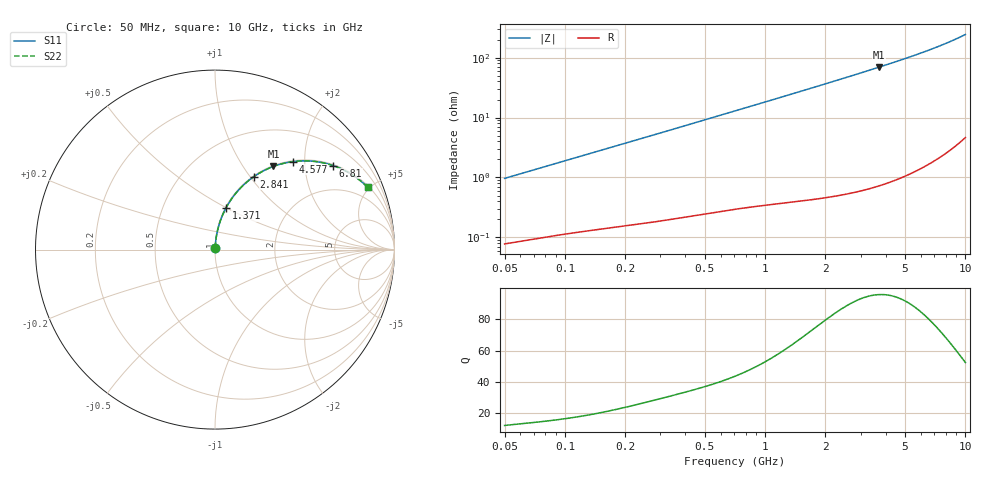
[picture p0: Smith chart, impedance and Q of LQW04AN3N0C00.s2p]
!Murata Part Number: LQW04AN3N0C00
!These Parameters are Measured in Series Mode Connection
!  o--[Z]--o
!Port1  Port2
!  o-------o
!Freq. Start=50[MHz] Stop=10[GHz], 401[Steps]
# Hz S RI R 50
!Freq.(Hz)	S 11(Real)	S 11(Imag)	S 21(Real)	S 21(Imag)	S 12(Real)	S 12(Imag)	S 22(Real)	S 22(Imag)
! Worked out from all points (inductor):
!   401 points, 50 MHz to 10 GHz, reference 50 ohm
!   read as one part in series: L = 3.04 nH near 51.34 MHz
!   highest Q = 95.6 at 3.703 GHz (marker M1), where L = 2.97 nH
!   S11 on the Smith chart (normalised r, x): 50 MHz: 1.00, +0.02; 1.371 GHz: 1.01, +0.50; 2.841 GHz: 1.01, +1.05; 4.577 GHz: 1.02, +1.74; 6.81 GHz: 1.04, +2.79; 10 GHz: 1.09, +4.86
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5e7  0.000871 0.00961  0.9991 -0.00961  0.9991 -0.00961  0.000871 0.00961
5.134228e7  0.000887 0.00986  0.9991 -0.00986  0.9991 -0.00986  0.000887 0.00986
1.214486e8  0.00176 0.0227  0.9982 -0.0227  0.9982 -0.0227  0.00176 0.0227
1.956524e8  0.00284 0.0361  0.9972 -0.0361  0.9972 -0.0361  0.00284 0.0361
2.949953e8  0.00479 0.054  0.9952 -0.054  0.9952 -0.054  0.00479 0.054
4.689809e8  0.00964 0.0848  0.9904 -0.0848  0.9904 -0.0848  0.00964 0.0848
7.071068e8  0.0191 0.126  0.9809 -0.126  0.9809 -0.126  0.0191 0.126
9.978194e8  0.0349 0.1744  0.9651 -0.1744  0.9651 -0.1744  0.0349 0.1744
1.371241e9  0.0617 0.2329  0.9383 -0.2329  0.9383 -0.2329  0.0617 0.2329
1.717543e9  0.0922 0.2825  0.9078 -0.2825  0.9078 -0.2825  0.0922 0.2825
2.23851e9  0.1464 0.3476  0.8536 -0.3476  0.8536 -0.3476  0.1464 0.3476
2.841223e9  0.2175 0.4071  0.7825 -0.4071  0.7825 -0.4071  0.2175 0.4071
3.243629e9  0.2676 0.4374  0.7324 -0.4374  0.7324 -0.4374  0.2676 0.4374
3.703027e9  0.3255 0.4634  0.6745 -0.4634  0.6745 -0.4634  0.3255 0.4634
4.171863e9  0.3839 0.4811  0.6161 -0.4811  0.6161 -0.4811  0.3839 0.4811
4.577181e9  0.4327 0.4902  0.5673 -0.4902  0.5673 -0.4902  0.4327 0.4902
5.583245e9  0.5445 0.4924  0.4555 -0.4924  0.4555 -0.4924  0.5445 0.4924
6.207365e9  0.6056 0.4827  0.3944 -0.4827  0.3944 -0.4827  0.6056 0.4827
6.810442e9  0.6585 0.4678  0.3415 -0.4678  0.3415 -0.4678  0.6585 0.4678
8.198065e9  0.7585 0.4205  0.2415 -0.4205  0.2415 -0.4205  0.7585 0.4205
9.359165e9  0.822 0.3739  0.178 -0.3739  0.178 -0.3739  0.822 0.3739
1e10  0.8506 0.3471  0.1494 -0.3471  0.1494 -0.3471  0.8506 0.3471
